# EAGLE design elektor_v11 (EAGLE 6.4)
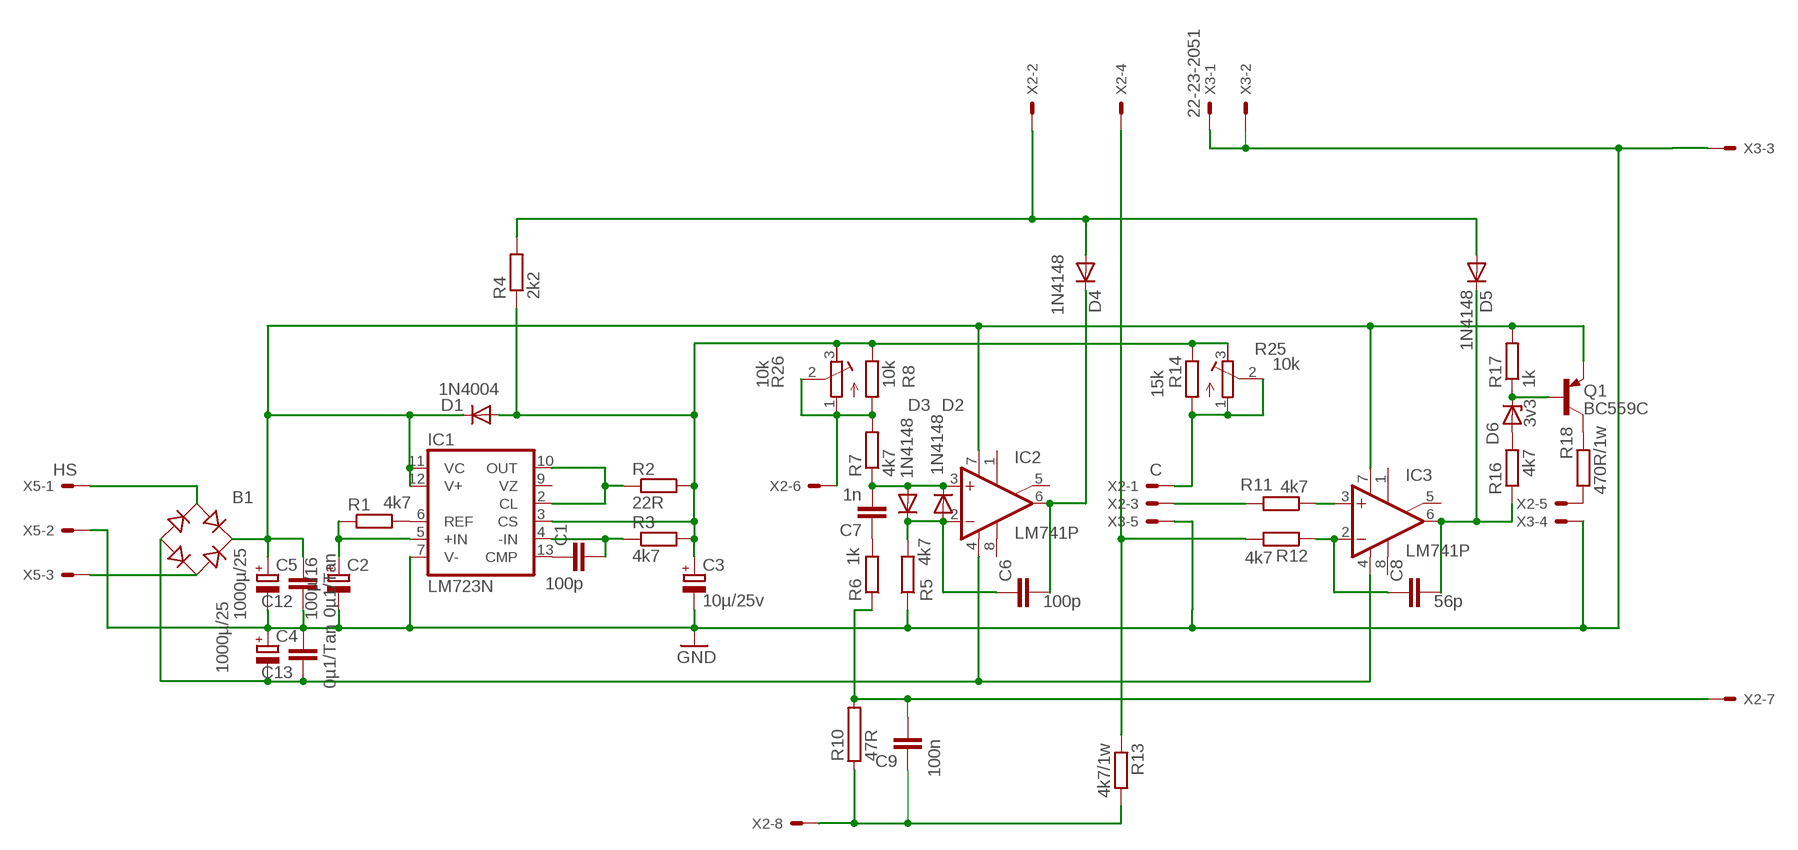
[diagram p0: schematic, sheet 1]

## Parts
B1  RB1A  [RB1A]
C1  100p  C-EU025-024X044  [C025-024X044]
C2  100µ/16  CPOL-EUE2.5-6  [E2,5-6]
C3  10µ/25v  CPOL-EUE2.5-6  [E2,5-6]
C4  1000µ/25  CPOL-EUE5-13  [E5-13]
C5  1000µ/25  CPOL-EUE5-13  [E5-13]
C6  100p  C-EU050-024X044  [C050-024X044]
C7  1n  C-EU050-024X044  [C050-024X044]
C8  56p  C-EU050-024X044  [C050-024X044]
C9  100n  C-EU025-024X044  [C025-024X044]
C12  0µ1/Tan  C-EU025-024X044  [C025-024X044]
C13  0µ1/Tan  C-EU025-024X044  [C025-024X044]
D1  1N4004  [DO41-10]
D2  1N4148  1N4148DO35-7  [DO35-7]
D3  1N4148  1N4148DO35-7  [DO35-7]
D4  1N4148  1N4148DO35-7  [DO35-7]
D5  1N4148  1N4148DO35-7  [DO35-7]
D6  3v3  ZENER-DIODEDO34-7  [DO34Z7]
IC1  LM723N  [DIL14]
IC2  LM741P  [DIL08]
IC3  LM741P  [DIL08]
Q1  BC559C  [TO92-EBC]
R1  4k7  R-EU_0207/2V  [0207/2V]
R2  22R  R-EU_0207/2V  [0207/2V]
R3  4k7  R-EU_0207/2V  [0207/2V]
R4  2k2  R-EU_0204/7  [0204/7]
R5  4k7  R-EU_0207/2V  [0207/2V]
R6  1k  R-EU_0204/7  [0204/7]
R7  4k7  R-EU_0207/5V  [0207/5V]
R8  10k  R-EU_0207/2V  [0207/2V]
R10  47R  RKH218-8  [KH218-8]
R11  4k7  R-EU_0207/12  [0207/12]
R12  4k7  R-EU_0204/7  [0204/7]
R13  4k7/1w  R-EU_0204/7  [0204/7]
R14  15k  R-EU_0207/2V  [0207/2V]
R16  4k7  R-EU_0207/5V  [0207/5V]
R17  1k  R-EU_0207/5V  [0207/5V]
R18  470R/1w  R-EU_0204/7  [0204/7]
R25  10k  R-TRIMM64Y  [RTRIM64Y]
R26  10k  R-TRIMM64Y  [RTRIM64Y]
X2  C  22-23-2081  [22-23-2081]
X3  22-23-2051  [22-23-2051]
X5  HS  22-23-2031  [22-23-2031]

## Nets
GND: C2.- C3.- C4.+ C5.- C12.1 C13.2 IC1.7(V-) R5.1 X3.1 X3.2 X3.3 X3.4 X3.5 X5.2
N$1: IC1.6(REF) R1.2
N$2: C2.+ IC1.5(+IN) R1.1
N$3: C1.1 IC1.13(CMP)
N$4: C1.2 IC1.4(-IN) R3.1
N$5: IC1.2(CL) IC1.10(OUT) R2.1
N$6: R12.2 R13.1 X2.4
N$7: C6.1 D2.A D3.C IC2.2(-IN) R5.2
N$8: R18.1 X2.5
N$9: C7.2 D2.C D3.A IC2.3(+IN) R7.1
N$10: C6.2 D4.C IC2.6(OUT)
N$11: C9.1 R10.1 R13.2 X2.8
N$12: B1.AC1 X5.1
N$13: B1.AC2 X5.3
N$14: B1.+ C5.+ C12.2 D1.C IC1.11(VC) IC1.12(V+) IC2.7(V+) IC3.7(V+) Q1.E R17.2
N$15: B1.- C4.- C13.1 IC2.4(V-) IC3.4(V-)
N$16: C7.1 R6.2
N$17: R7.2 R8.1 R26.1(A) R26.2(S) X2.6
N$18: C3.+ D1.A IC1.3(CS) R2.2 R3.2 R4.1 R8.2 R14.2 R25.3(E) R26.3(E)
N$19: C9.2 R6.1 R10.2 X2.7
N$21: C8.2 D5.C IC3.6(OUT) R16.1
N$22: C8.1 IC3.2(-IN) R12.1
N$25: R11.2 X2.3
N$26: R14.1 R25.1(A) R25.2(S) X2.1
N$28: IC3.3(+IN) R11.1
N$29: D6.A R16.2
N$30: D6.C Q1.B R17.1
N$31: Q1.C R18.2
N$34: D4.A D5.A R4.2 X2.2
Unconnected: IC1.9(VZ) IC2.1(ON1) IC2.5(ON2) IC2.8(OPT) IC3.1(ON1) IC3.5(ON2) IC3.8(OPT)

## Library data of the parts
B1 = rectifier:RB1A: RECTIFIER 1 A
C1 C6-C9 C12 C13 = rcl:C-EU: CAPACITOR, European symbol
C2-C5 = rcl:CPOL-EU: POLARIZED CAPACITOR, European symbol
D1 = diode:1N4004: DIODE
D2-D5 = diode:1N4148: DIODE
D6 = diode:ZENER-DIODE: Z-Diode
IC1 = linear:*723: Positive VOLTAGE REGULATOR
IC2 IC3 = linear:*741: OP AMP
Q1 = transistor-pnp:BC559*: PNP Transistror
R1-R8 R11-R14 R16-R18 = rcl:R-EU_: RESISTOR, European symbol
R10 = resistor-power:R: Power Resitor; OC_FARNELL: unknown; OC_NEWARK: unknown
R25 R26 = rcl:R-TRIMM: Trimm resistor
X2 = con-molex:22-23-2081: .100" (2.54mm) Center Header - 8 Pin; MF: MOLEX; MPN: 22-23-2081; OC_FARNELL: 1756826; OC_NEWARK: 01C7592
X3 = con-molex:22-23-2051: .100" (2.54mm) Center Header - 5 Pin; MF: MOLEX; MPN: 22-23-2051; OC_FARNELL: 1462952; OC_NEWARK: 38C9178
X5 = con-molex:22-23-2031: .100" (2.54mm) Center Header - 3 Pin; MF: MOLEX; MPN: 22-23-2031; OC_FARNELL: 1462950; OC_NEWARK: 30C0862

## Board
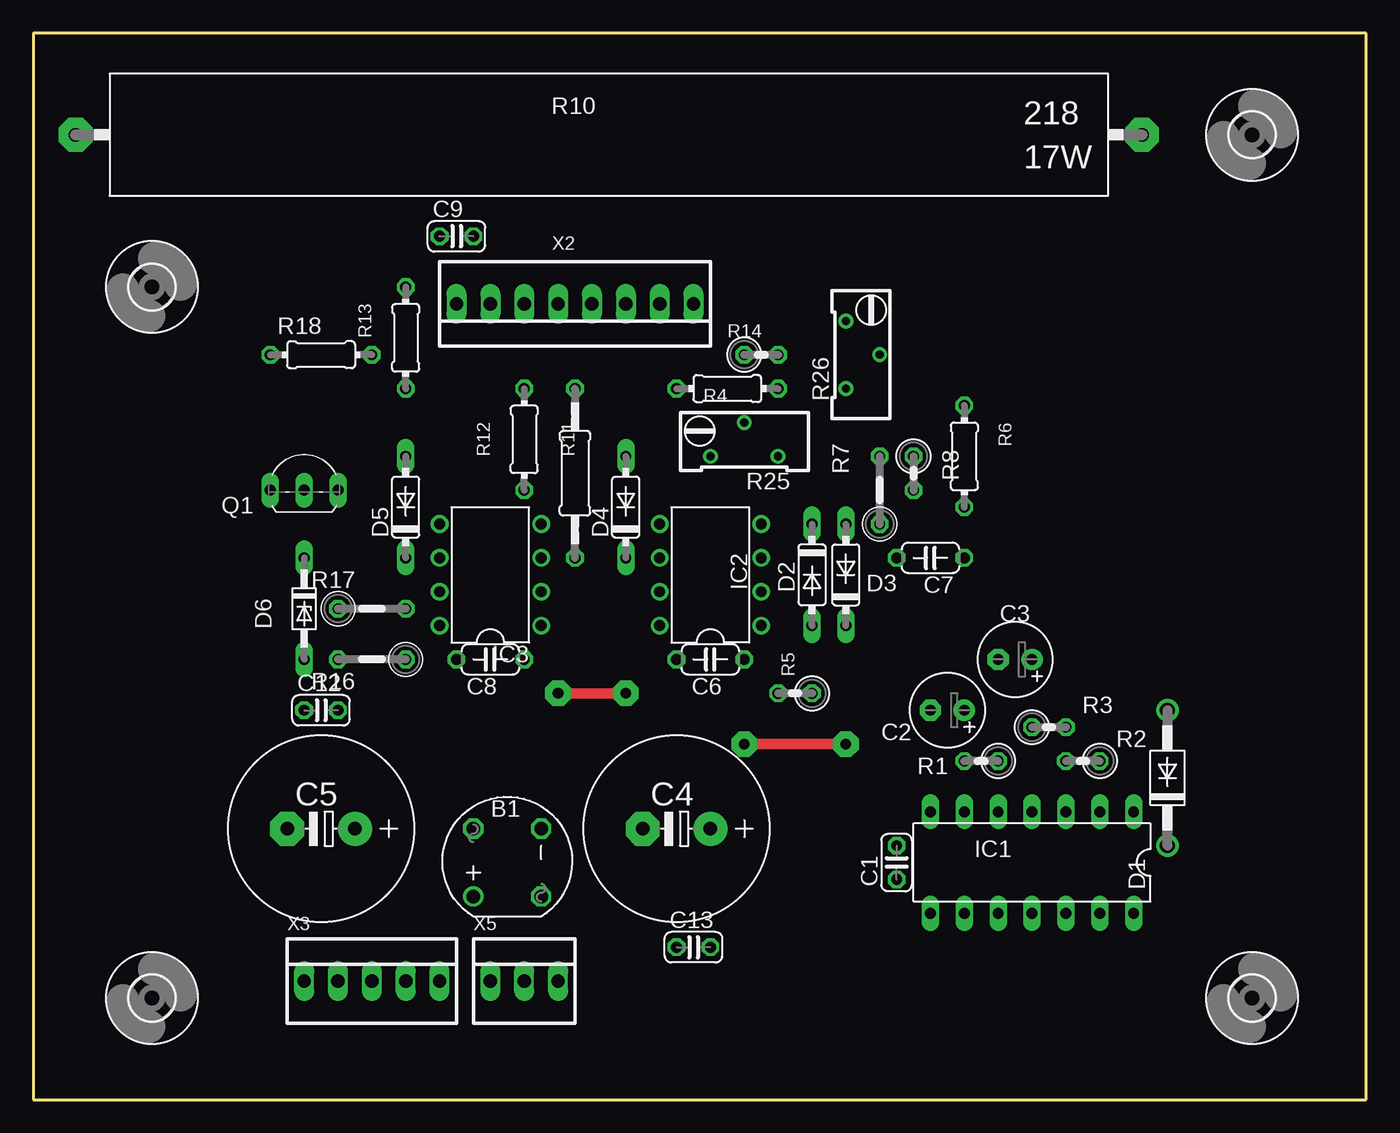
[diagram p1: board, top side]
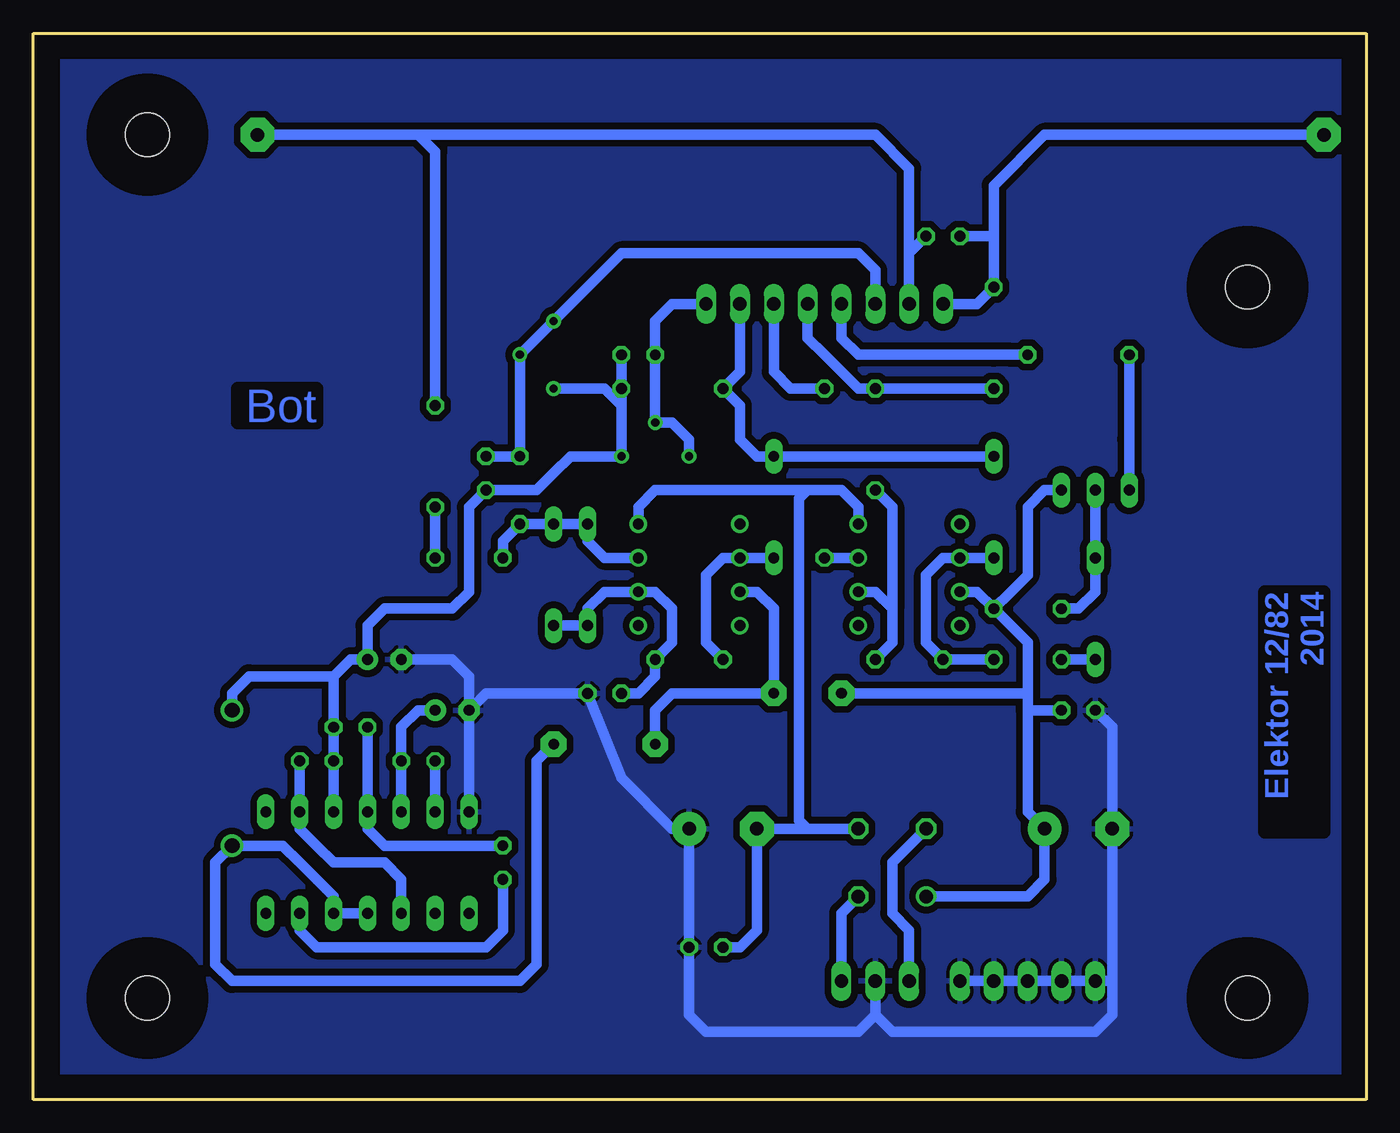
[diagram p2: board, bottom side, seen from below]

Size 100 x 80 mm. Coordinates in mm from the lower left corner, seen from the top.
Outline: 0,0 100,0 100,80 0,80 0,0
Copper layers (1*16): Top 0.035mm / dielectric 2.5mm / Bottom 0.035mm
Design rules "default *": minimum track width 12mil, minimum drill 24mil, track to track 10mil, track to pad 8mil, pad to pad 8mil, via to via 8mil, smd to smd 8mil, copper to edge 70mil, drill to drill 8mil, minimum pad ring 10mil, minimum via ring 8mil, stop-mask expansion 4mil, vias tented up to drill 0mil, thermal gap 10mil

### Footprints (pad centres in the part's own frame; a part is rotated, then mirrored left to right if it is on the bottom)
RB1A = drill 1.016: + -2.54,2.54 | drill 1.016 octagon: - 2.54,-2.54; AC1 2.54,2.54; AC2 -2.54,-2.54
C025-024X044 = drill 0.813 octagon: 1 -1.27,0; 2 1.27,0
E2,5-6 = drill 0.813 pad 1.6: + -1.27,0 | drill 0.813 pad 1.6 octagon: - 1.27,0
E5-13 = drill 1.016 pad 2.54: + -2.54,0 | drill 1.016 pad 2.54 octagon: - 2.54,0
C050-024X044 = drill 0.813 octagon: 1 -2.54,0; 2 2.54,0
DO41-10 = drill 1.118: A 5.08,0; C -5.08,0
DO35-7 = drill 0.813 long: A 3.81,0; C -3.81,0
DO34Z7 = drill 0.813 long: A 3.81,0; C -3.81,0
DIL14 = drill 0.813 long: 1 -7.62,-3.81; 2 -5.08,-3.81; 3 -2.54,-3.81; 4 0,-3.81; 5 2.54,-3.81; 6 5.08,-3.81; 7 7.62,-3.81; 8 7.62,3.81; 9 5.08,3.81; 10 2.54,3.81; 11 0,3.81; 12 -2.54,3.81; 13 -5.08,3.81; 14 -7.62,3.81
DIL08 = drill 0.813 pad 1.27: 1 -3.81,-3.81; 2 -1.27,-3.81; 3 1.27,-3.81; 4 3.81,-3.81; 5 3.81,3.81; 6 1.27,3.81; 7 -1.27,3.81; 8 -3.81,3.81
TO92-EBC = drill 0.813 long: B 0,-1.27; C -2.54,-1.27; E 2.54,-1.27
0207/2V = drill 0.813 octagon: 1 -1.27,0; 2 1.27,0
0204/7 = drill 0.813 octagon: 1 -3.81,0; 2 3.81,0
0207/5V = drill 0.813 octagon: 1 -2.54,0; 2 2.54,0
KH218-8 = drill 1.016 pad 2.54 octagon: 1 -40.005,0; 2 40.005,0
0207/12 = drill 0.813 octagon: 1 -6.35,0; 2 6.35,0
RTRIM64Y = drill 0.61: 1 0,-2.54; 2 -2.54,0; 3 0,2.54
3,3 = hole 3.3: 0,0
22-23-2081 = drill 1 long: 1 -8.89,0; 2 -6.35,0; 3 -3.81,0; 4 -1.27,0; 5 1.27,0; 6 3.81,0; 7 6.35,0; 8 8.89,0
22-23-2051 = drill 1 long: 1 -5.08,0; 2 -2.54,0; 3 0,0; 4 2.54,0; 5 5.08,0
22-23-2031 = drill 1 long: 1 -2.54,0; 2 0,0; 3 2.54,0

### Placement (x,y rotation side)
B1  35.56,17.78 90 top
C1  64.77,17.78 90 top
C2  68.58,29.21 180 top
C3  73.66,33.02 180 top
C4  48.26,20.32 180 top
C5  21.59,20.32 180 top
C6  50.8,33.02 180 top
C7  67.31,40.64 180 top
C8  34.29,33.02 180 top
C9  31.75,64.77 0 top
C12  21.59,29.21 0 top
C13  49.53,11.43 0 top
D1  85.09,24.13 90 top
D2  58.42,39.37 270 top
D3  60.96,39.37 90 top
D4  44.45,44.45 90 top
D5  27.94,44.45 90 top
D6  20.32,36.83 270 top
IC1  74.93,17.78 180 top
IC2  50.8,39.37 90 top
IC3  34.29,39.37 90 top
Q1  20.32,46.99 0 top
R1  71.12,25.4 180 top
R2  78.74,25.4 180 top
R3  76.2,27.94 0 top
R4  52.07,53.34 180 top
R5  57.15,30.48 180 top
R6  69.85,48.26 270 top
R7  63.5,45.72 90 top
R8  66.04,46.99 270 top
R10  43.18,72.39 0 top
R11  40.64,46.99 90 top
R12  36.83,49.53 90 top
R13  27.94,57.15 90 top
R14  54.61,55.88 0 top
R16  25.4,33.02 180 top
R17  25.4,36.83 0 top
R18  21.59,55.88 180 top
R25  53.34,48.26 270 top
R26  60.96,55.88 180 top
U$1  [3,3]  8.89,7.62 0 top
U$2  [3,3]  91.44,7.62 0 top
U$3  [3,3]  8.89,60.96 0 top
U$4  [3,3]  91.44,72.39 0 top
X2  40.64,59.69 180 top
X3  25.4,8.89 0 top
X5  36.83,8.89 0 top

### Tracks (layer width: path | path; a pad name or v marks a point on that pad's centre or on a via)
GND
  Bottom 0.8: 19.05,8.89 19.05,10.16 C5.- 19.05,27.94 C12.1 | C3.- 68.58,33.02 67.31,31.75 C2.- | C2.- IC1.7 | C2.- 66.04,30.48 R5.1 55.88,24.13 54.61,22.86 53.34,21.59 52.07,20.32 C4.+ C13.2 50.8,6.35 49.53,5.08 38.1,5.08 36.83,6.35 | X3.5 X3.4 X3.3 X3.2 X3.1 19.05,8.89 | 36.83,6.35 X5.2 36.83,6.35 | 36.83,6.35 35.56,5.08 31.75,5.08 30.48,5.08 20.32,5.08 19.05,6.35 19.05,8.89
  pour Bottom (isolate 0.5): 1.27,1.27 1.27,78.74 97.79,78.74 97.79,1.27
N$1
  Bottom 0.8: IC1.6 R1.2
N$2
  Bottom 0.8: C2.+ 71.12,29.21 72.39,27.94 R1.1 IC1.5
N$3
  Bottom 0.8: IC1.13 80.01,12.7 78.74,11.43 66.04,11.43 64.77,12.7 C1.1
N$4
  Bottom 0.8: R3.1 IC1.4 74.93,20.32 73.66,19.05 C1.2
N$5
  Bottom 0.8: R2.1 IC1.2 80.01,20.32 78.74,19.05 77.47,17.78 73.66,17.78 72.39,16.51 IC1.10
N$6
  Bottom 0.8: R13.1 R12.2 38.1,53.34 40.64,55.88 41.91,57.15 X2.4
N$7
  Bottom 0.8: D3.C D2.A 58.42,36.83 57.15,38.1 IC2.2 53.34,38.1 52.07,36.83 52.07,34.29 C6.1 53.34,31.75 54.61,30.48 R5.2
N$8
  Bottom 0.8: X2.5 39.37,57.15 38.1,55.88 27.94,55.88 26.67,55.88 R18.1
N$9
  Bottom 0.8: IC2.3 57.15,40.64 58.42,41.91 D2.C D3.A R7.1 64.77,41.91 C7.2
N$10
  Bottom 0.8: C6.2 49.53,34.29 49.53,39.37 48.26,40.64 IC2.6 D4.C
N$11
  Bottom 0.8: R10.1 24.13,72.39 27.94,68.58 27.94,64.77 | 27.94,64.77 R13.2 29.21,59.69 X2.8 | C9.1 27.94,64.77
N$12
  Bottom 0.8: B1.AC1 35.56,17.78 35.56,13.97 34.29,12.7 34.29,11.43 X5.1
N$13
  Bottom 0.8: X5.3 39.37,13.97 B1.AC2
N$14  (via drill 0.8 pad 1.93)
  Top 0.8: v44.45,30.48 v39.37,30.48 | v53.34,26.67 v60.96,26.67
  Bottom 0.8: B1.+ 25.4,15.24 24.13,16.51 C5.+ 25.4,21.59 25.4,29.21 | IC3.7 29.21,38.1 R17.2 | Q1.E 24.13,45.72 25.4,44.45 25.4,39.37 26.67,38.1 R17.2 | R17.2 25.4,34.29 25.4,30.48 | 25.4,30.48 25.4,29.21 | IC1.11 IC1.12 77.47,15.24 80.01,17.78 81.28,19.05 D1.C 86.36,17.78 86.36,10.16 85.09,8.89 63.5,8.89 62.23,10.16 62.23,25.4 v60.96,26.67 | IC2.7 45.72,38.1 44.45,36.83 v44.45,30.48 52.07,30.48 53.34,29.21 v53.34,26.67 | v39.37,30.48 25.4,30.48 | C12.2 25.4,29.21
N$15
  Bottom 0.8: B1.- 41.91,20.32 | 41.91,20.32 C4.- 45.72,12.7 46.99,11.43 C13.1 | IC2.4 54.61,44.45 53.34,45.72 41.91,45.72 | 41.91,45.72 39.37,45.72 38.1,44.45 IC3.4 | 41.91,45.72 42.55,45.09 42.55,20.95 41.91,20.32
N$16
  Bottom 0.8: R6.2 C7.1
N$17
  Bottom 0.8: R8.1 R7.2 R26.2 R26.1 55.88,63.5 38.1,63.5 36.83,62.23 X2.6
N$18
  Bottom 0.8: 55.88,52.07 R4.1 R14.2 | 55.88,52.07 55.88,49.53 R25.3 58.42,48.26 59.69,48.26 60.96,46.99 62.23,45.72 63.5,45.72 | R26.3 57.15,53.34 55.88,52.07 | 63.5,45.72 64.77,45.72 | R8.2 64.77,45.72 | 64.77,45.72 63.5,45.72 | 64.77,45.72 R8.2 | 77.47,31.75 76.2,33.02 C3.+ 74.93,35.56 73.66,36.83 68.58,36.83 67.31,38.1 67.31,44.45 R8.2 | 77.47,31.75 R3.2 R2.2 IC1.3 | D1.A 85.09,30.48 83.82,31.75 77.47,31.75
N$19
  Bottom 0.8: X2.7 34.29,63.5 | 34.29,63.5 34.29,64.77 34.29,69.85 36.83,72.39 71.12,72.39 | C9.2 34.29,63.5 | 71.12,72.39 R10.2 | R6.1 69.85,71.12 71.12,72.39
N$21
  Bottom 0.8: R16.1 C8.2 33.02,34.29 33.02,39.37 31.75,40.64 IC3.6 D5.C
N$22
  Bottom 0.8: C8.1 35.56,34.29 35.56,36.83 | 35.56,36.83 36.83,38.1 IC3.2 | R12.1 35.56,44.45 35.56,36.83
N$25
  Bottom 0.8: X2.3 44.45,54.61 43.18,53.34 R11.2
N$26
  Bottom 0.8: R25.1 50.8,49.53 52.07,50.8 R25.2 R14.1 53.34,58.42 52.07,59.69 X2.1
N$28
  Bottom 0.8: R11.1 IC3.3
N$29
  Bottom 0.8: D6.A R16.2
N$30
  Bottom 0.8: Q1.B D6.C 20.32,38.1 21.59,36.83 R17.1
N$31
  Bottom 0.8: R18.2 17.78,49.53 Q1.C
N$34
  Bottom 0.8: D5.A D4.A 45.72,48.26 46.99,49.53 46.99,52.07 R4.2 46.99,54.61 X2.2

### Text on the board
Bottom: Bot | Elektor 12/82 / 2014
